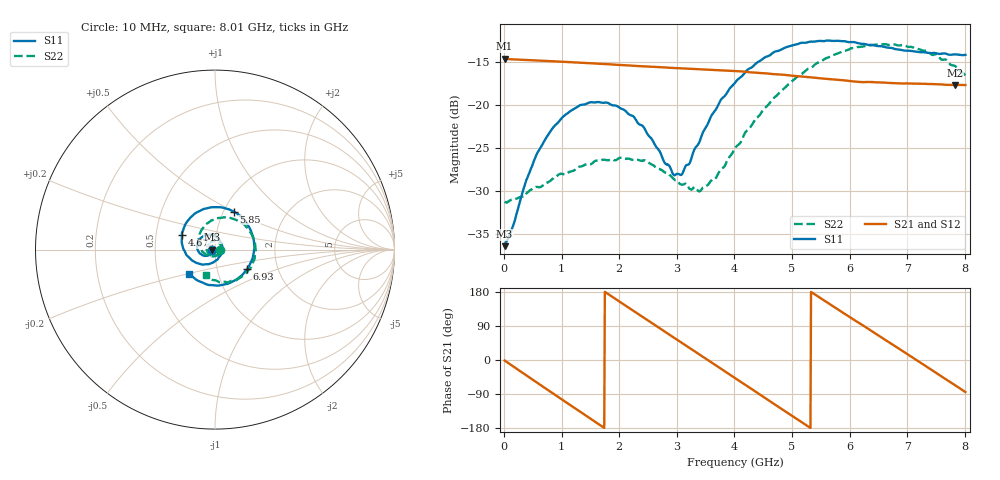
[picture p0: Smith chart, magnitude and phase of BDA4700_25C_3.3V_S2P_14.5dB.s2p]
!Agilent Technologies,E5071B,MY42404982,A.09.10
!Date: Mon Oct 20 18:09:07 2025
!Data & Calibration Information:
!Freq	S11:SOLT2(ON)	S21:SOLT2(ON)	S12:SOLT2(ON)	S22:SOLT2(ON)
# Hz S RI R 50
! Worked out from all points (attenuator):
!   801 points, 10 MHz to 8.01 GHz, reference 50 ohm
!   highest |S21| = -14.59 dB at 10 MHz (marker M1); lowest = -17.7 dB at 7.83 GHz (marker M2)
!   lowest |S11| = -36.5 dB at 10 MHz (marker M3), VSWR 1.03, Z = 48.5 - j0.124 ohm
!   |S11| at or under -10 dB: start of sweep to end of sweep
!   |S22| runs from -31.4 to -12.9 dB; largest |S21 - S12| = 0.0022
!   S11 on the Smith chart (normalised r, x): 10 MHz: 0.97, -0.00; 4.67 GHz: 0.68, +0.11; 5.85 GHz: 1.11, +0.50; 6.93 GHz: 1.39, -0.32; 8.01 GHz: 0.73, -0.20
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1e7  -0.015 -0.00128  0.1863 -0.00409  0.1862 -0.0042  0.0272 -0.00101
6e8  -0.0415 -0.0346  0.0839 -0.1612  0.0837 -0.1613  0.0118 -0.0309
1.01e9  -0.0811 -0.0239  -0.0452 -0.1731  -0.0451 -0.173  -0.0194 -0.0346
1.35e9  -0.1 0.0101  -0.134 -0.1148  -0.134 -0.1148  -0.0415 -0.0142
1.71e9  -0.0872 0.0549  -0.1732 -0.0118  -0.1734 -0.0117  -0.0448 0.0171
2.08e9  -0.0455 0.0821  -0.1422 0.0947  -0.1423 0.0946  -0.0234 0.0426
2.42e9  0.00273 0.0746  -0.0632 0.1559  -0.0632 0.1558  0.00729 0.0468
2.68e9  0.0303 0.0459  0.0118 0.1661  0.0116 0.1659  0.0259 0.0336
2.94e9  0.0389 0.00598  0.0825 0.1424  0.0825 0.142  0.0346 0.0136
3.08e9  0.0353 -0.017  0.1145 0.117  0.1134 0.1177  0.0343 0.000248
3.41e9  0.000738 -0.063  0.1576 0.0359  0.1578 0.0358  0.0181 -0.026
3.67e9  -0.0454 -0.0816  0.1556 -0.0367  0.1556 -0.0372  -0.00611 -0.0368
4.01e9  -0.1174 -0.0664  0.1065 -0.1165  0.1067 -0.1162  -0.0466 -0.0307
4.67e9  -0.1849 0.0808  -0.062 -0.1382  -0.0616 -0.1386  -0.0914 0.059
5.35e9  -0.0575 0.227  -0.1447 0.00594  -0.1447 0.00501  -0.00559 0.1662
5.85e9  0.1035 0.2116  -0.0865 0.1098  -0.0863 0.1096  0.1201 0.1645
6.27e9  0.1985 0.1091  0.00534 0.1358  0.00746 0.1355  0.2041 0.0843
6.68e9  0.2134 -0.0314  0.0916 0.0986  0.0919 0.0984  0.2227 -0.0281
6.93e9  0.1778 -0.1086  0.1231 0.0516  0.1233 0.051  0.2021 -0.0968
7.41e9  0.0401 -0.1969  0.1204 -0.0556  0.1204 -0.0558  0.0971 -0.1731
7.83e9  -0.0965 -0.1725  0.0524 -0.1198  0.0523 -0.12  -0.0141 -0.1683
8.01e9  -0.1422 -0.1352  0.0122 -0.1302  0.0126 -0.1302  -0.0518 -0.1399
